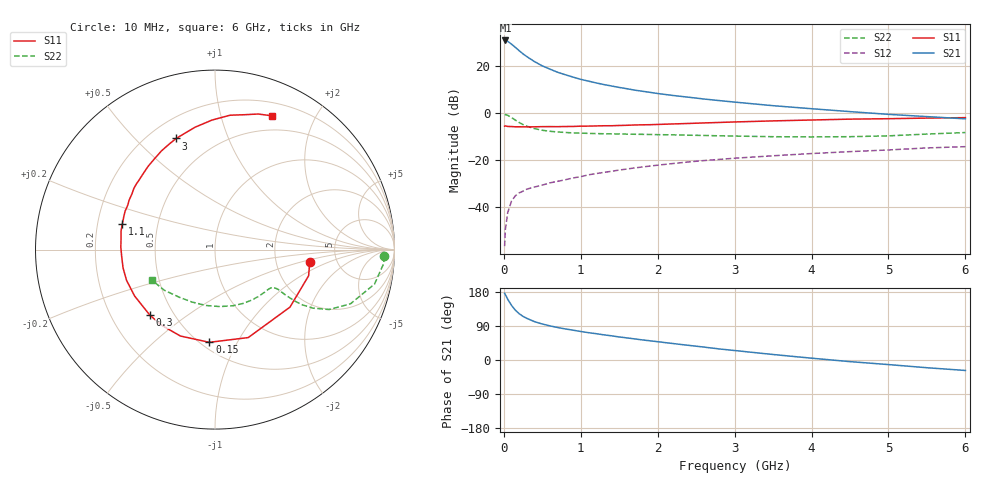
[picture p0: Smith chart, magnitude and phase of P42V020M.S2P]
! SIEMENS Small Signal Semiconductors
! BFP182
! Si NPN RF Bipolar Junction Transistor in SOT143
! VCE = 2 V  IC = 20 mA
! Common Emitter S-Parameters:  March  1996
# GHz  S  MA  R  50
!  f  S11  S21  S12  S22
! GHz  MAG  ANG  MAG  ANG  MAG  ANG  MAG  ANG
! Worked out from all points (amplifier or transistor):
!   36 points, 10 MHz to 6 GHz, reference 50 ohm
!   highest |S21| = 31.0 dB at 20 MHz (marker M1)
!   |S21| within 3 dB of that: start of sweep to 151.9 MHz
!   unconditionally stable (mu >= 1): 624 MHz to 5.662 GHz
!   at 250 MHz: K = 0.57, MSG = 29.2 dB, |S12| = -33.1 dB
!   at 1.4 GHz: K = 1.27, MAG = 15.0 dB, |S12| = -24.6 dB
!   at 6 GHz: K = 0.97, MSG = 5.9 dB, |S12| = -14.2 dB
!   S11 on the Smith chart (normalised r, x): 10 MHz: 3.14, -0.63; 150 MHz: 0.55, -0.78; 300 MHz: 0.37, -0.37; 1.1 GHz: 0.31, +0.12; 3 GHz: 0.31, +0.66; 6 GHz: 0.34, +1.46
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0.01  0.5326 -7.7  35.38 176.0  0.0015 85.3  0.9449 -2.3
0.02  0.5416 -15.6  35.46 172.3  0.0034 85.1  0.9421 -4.9
0.05  0.5265 -37.5  34.03 160.4  0.0077 79.1  0.9093 -12.2
0.1  0.5239 -69.3  29.58 144.1  0.0137 63.0  0.8131 -21.8
0.15  0.5176 -93.5  25.26 131.5  0.0177 56.6  0.7182 -27.7
0.2  0.5186 -111.8  21.47 122.1  0.0204 52.3  0.6376 -30.8
0.25  0.5158 -124.8  18.36 115.0  0.0222 50.0  0.5767 -32.3
0.3  0.5149 -134.7  16.04 109.8  0.0245 48.8  0.5324 -32.8
0.4  0.5172 -150.0  12.55 101.1  0.0272 48.9  0.4725 -32.8
0.5  0.5217 -160.9  10.22 95.0  0.0298 49.2  0.437 -32.5
0.6  0.5223 -168.7  8.697 90.0  0.0333 50.2  0.4154 -32.2
0.7  0.5213 -175.7  7.464 85.7  0.0359 51.6  0.4022 -32.5
0.8  0.5248 178.6  6.612 81.9  0.0388 52.7  0.3918 -32.8
1  0.5338 168.7  5.287 75.2  0.045 54.0  0.3794 -34.1
1.1  0.5356 164.4  4.841 72.1  0.0493 54.2  0.3748 -35.2
1.5  0.5522 150.1  3.555 60.8  0.0623 53.9  0.3645 -40.6
2.2  0.5953 128.7  2.399 43.4  0.0858 50.0  0.3491 -53.3
3  0.6561 109.3  1.735 25.0  0.1112 43.5  0.329 -71.7
3.5  0.6911 99.2  1.455 14.5  0.1253 39.1  0.3187 -84.9
4.5  0.7534 83.6  1.088 -4.3  0.1535 30.6  0.3191 -113.9
5.5  0.7929 72.3  0.853 -20.4  0.1839 22.1  0.3626 -141.5
6  0.8102 66.9  0.764 -27.6  0.1959 16.9  0.3909 -154.3
